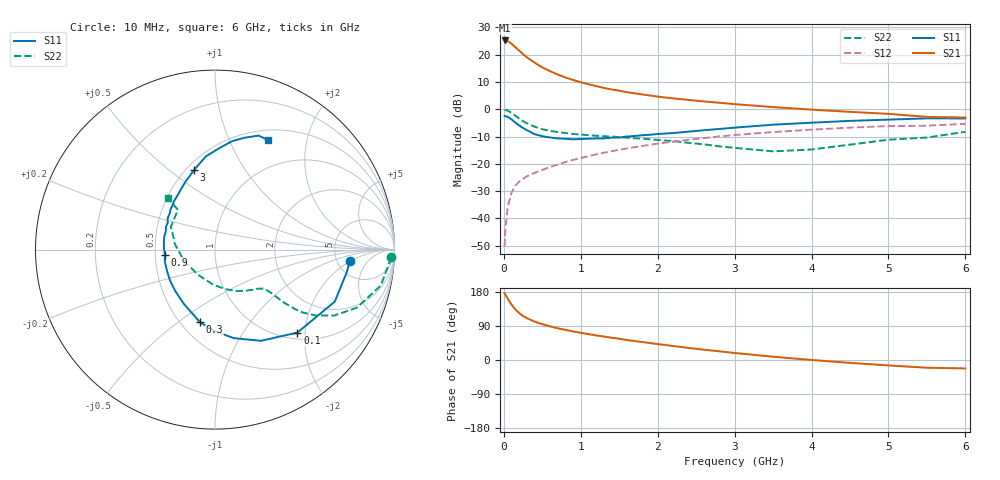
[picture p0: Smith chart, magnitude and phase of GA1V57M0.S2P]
! Infineon Technologies  Discrete & RF Semiconductors
! BF775
! Si NPN RF Bipolar Junction Transistor in SOT23
! VCE = 1.5 V  IC = 7 mA
! Common Emitter S-Parameters:  May  1996
# GHz  S  MA  R  50
!  f  S11  S21  S12  S22
! GHz  MAG  ANG  MAG  ANG  MAG  ANG  MAG  ANG
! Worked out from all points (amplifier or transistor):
!   36 points, 10 MHz to 6 GHz, reference 50 ohm
!   highest |S21| = 25.2 dB at 10 MHz (marker M1)
!   |S21| within 3 dB of that: start of sweep to 170.9 MHz
!   unconditionally stable (mu >= 1): 626.3 MHz to 4.287 GHz; 5.181 GHz to end of sweep
!   at 250 MHz: K = 0.60, MSG = 22.9 dB, |S12| = -25.5 dB
!   at 1.4 GHz: K = 1.15, MAG = 9.0 dB, |S12| = -15.4 dB
!   at 6 GHz: K = 1.00, MAG = 0.8 dB, |S12| = -5.4 dB
!   S11 on the Smith chart (normalised r, x): 10 MHz: 6.50, -1.98; 100 MHz: 1.14, -1.83; 300 MHz: 0.62, -0.61; 900 MHz: 0.56, -0.04; 3 GHz: 0.55, +0.62; 6 GHz: 0.62, +1.40
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0.01  0.7536 -5.0  18.2 176.3  0.0031 85.7  0.9827 -2.5
0.02  0.7448 -9.8  18.02 172.4  0.0065 86.3  0.9715 -4.9
0.05  0.7274 -23.5  17.65 161.8  0.0162 77.9  0.9454 -12.2
0.1  0.6516 -45.2  15.85 146.2  0.0296 69.3  0.8548 -22.2
0.15  0.5693 -63.2  13.67 133.2  0.0399 62.7  0.7599 -28.9
0.2  0.5041 -78.1  11.86 123.6  0.047 59.1  0.6727 -33.1
0.25  0.4526 -90.7  10.22 116.1  0.053 57.5  0.603 -35.6
0.3  0.4134 -101.6  8.944 110.2  0.059 56.3  0.5531 -36.7
0.4  0.3491 -119.7  7.136 101.5  0.0683 56.2  0.4787 -37.6
0.5  0.3201 -133.7  5.836 94.4  0.0774 57.0  0.4303 -37.6
0.6  0.3039 -145.6  4.977 88.8  0.0874 57.7  0.4025 -37.6
0.7  0.292 -156.5  4.329 83.8  0.097 58.2  0.3817 -37.8
0.9  0.281 -174.1  3.434 75.5  0.1179 58.5  0.3523 -38.5
1.1  0.2881 171.6  2.871 68.4  0.1382 58.5  0.3345 -40.7
1.3  0.2919 160.1  2.46 61.9  0.1597 57.5  0.3202 -43.1
1.6  0.3168 146.2  2.053 52.7  0.1913 55.5  0.301 -48.3
2.2  0.3658 125.1  1.58 37.0  0.2551 49.7  0.2607 -62.4
3  0.4595 104.6  1.241 18.5  0.3365 40.0  0.1959 -92.9
3.5  0.5213 95.7  1.095 8.7  0.3814 33.3  0.1693 -124.2
4.5  0.612 81.0  0.895 -7.6  0.4607 19.8  0.2246 172.6
5.5  0.6804 69.0  0.725 -20.4  0.4992 5.6  0.3027 133.1
6  0.6776 64.2  0.704 -22.3  0.5396 1.6  0.3858 132.4
